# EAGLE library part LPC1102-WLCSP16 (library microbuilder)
NXP Semiconductors LPC1102 microcontroller ARM 32-bit Cortex-M0 Microcontroller with MPU CPU clock up to 50MHz 32KByte on-chip Flash ROM with In-System Programming (ISP) and In-Application Programming (IAP) via On-Chip Bootloader 8KByte SRAM Nested Vectored Interrupt Controller SPI controller UART with full Modem Interface and RS485 Support 4 Timers with 4 capture channels and 13 output channels Watchdog (WDT) Sytem tick timer 10-bit ADC with 5 channels Power Management Unit (PMU) Brownout detection 12MHz internal RC oscillator Serial Wire Debug/Trace port
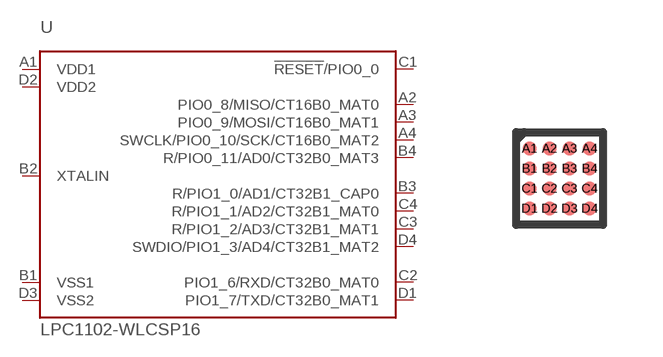
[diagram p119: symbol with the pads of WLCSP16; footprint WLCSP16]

Designator prefix -

## LPC1102-WLCSP16  [WLCSP16]
A1  VDD1  pwr
A2  PIO0_8/MISO/CT16B0_MAT0
A3  PIO0_9/MOSI/CT16B0_MAT1
A4  SWCLK/PIO0_10/SCK/CT16B0_MAT2
B1  VSS1  pwr
B2  XTALIN  pas
B3  R/PIO1_0/AD1/CT32B1_CAP0
B4  R/PIO0_11/AD0/CT32B0_MAT3
C1  !RESET!/PIO0_0
C2  PIO1_6/RXD/CT32B0_MAT0
C3  R/PIO1_2/AD3/CT32B1_MAT1
C4  R/PIO1_1/AD2/CT32B1_MAT0
D1  PIO1_7/TXD/CT32B0_MAT1
D2  VDD2  pwr
D3  VSS2  pwr
D4  SWDIO/PIO1_3/AD4/CT32B1_MAT2

## Footprint WLCSP16 (pad centres in mm)
WLCSP-16 2.17x3.32x0.6mm Wafer Level chip-size package
smd 0.35 x 0.35: A1 -0.75,0.75; A2 -0.25,0.75; A3 0.25,0.75; A4 0.75,0.75; B1 -0.75,0.25; B2 -0.25,0.25; B3 0.25,0.25; B4 0.75,0.25; C1 -0.75,-0.25; C2 -0.25,-0.25; C3 0.25,-0.25; C4 0.75,-0.25; D1 -0.75,-0.75; D2 -0.25,-0.75; D3 0.25,-0.75; D4 0.75,-0.75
